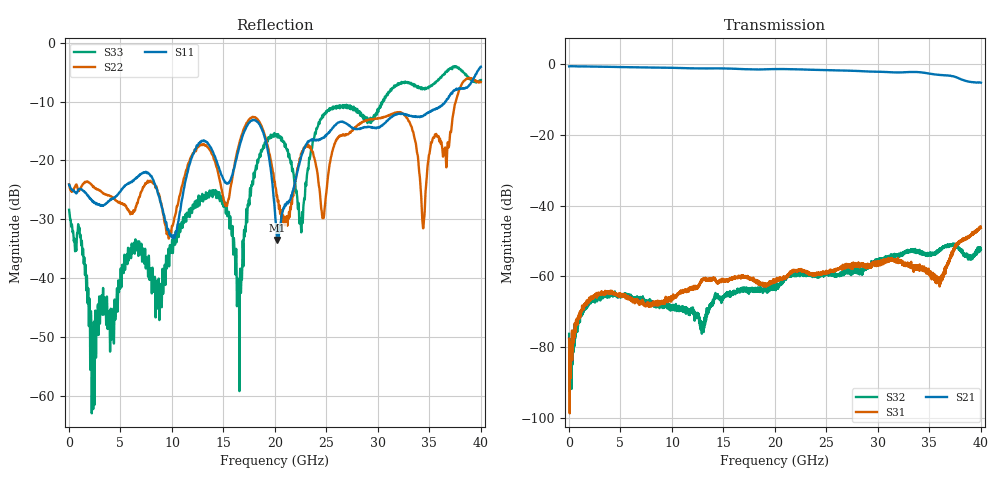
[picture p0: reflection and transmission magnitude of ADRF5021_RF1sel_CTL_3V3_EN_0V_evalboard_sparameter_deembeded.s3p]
! Device:  ADRF5021
! Description: SOI MMIC SPDT Non-Reflective Switch
! Frequency:  9 kHz -  30 GHz
! Ports:
! 	RFC	= Port 1
!	RF1	= Port 2
!	RF2	= Port 3
! Vdd:  +3.3 Volt
! Vss:  -2.5 Volt
! Control:  0/+3.3 Volt
! State:  RF1 Selected (Vctl= 3.3 V, Ven= 0 V)
! Data:	Data was collected using a calibrated network analyzer with AFR software.
!	Fixtures were calculated using AFR and fixturing was applied to collect
!	this Deembedded  S Parameter data of ADRF5021.
! Note:	Analog Devices supplies this data as a sample of measured data at the package pin
!	for this product.  Your particular data for this product may vary.
!	Data was taken at 25 degrees C.
!	Analog Devices reserves the right to change this data at anytime.
# Hz S  dB  R 50
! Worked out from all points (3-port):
!   4000 points, 10 MHz to 40 GHz, reference 50 ohm
!   strongest paths, dB at 10 MHz, 10.01 GHz, 20.01 GHz, 30.01 GHz, 40 GHz:
!     S21: -0.7, -1.1, -1.4, -2.2, -5.3
!     S31: -77.6, -66.2, -61.0, -56.4, -46.3
!     S32: -76.2, -68.1, -63.7, -55.7, -52.3
!   lowest |S11| = -33.5 dB at 20.24 GHz (marker M1), VSWR 1.04, Z = 48 + j0.696 ohm
!   |S11| at or under -10 dB: start of sweep to 36.54 GHz
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1e7  -24.09 -1.8  -0.68 -0.2  -82.91 -11.9
     -0.68 -0.1  -24.04 -2.1  -77.96 -98.2
     -77.58 63.8  -76.18 166.8  -28.37 -165.7
2.35e9  -26.90 -40.8  -0.74 -28.0  -65.82 54.0
        -0.75 -27.9  -24.50 -36.0  -66.67 35.7
        -65.82 52.2  -66.93 36.6  -62.18 -25.7
1.369e10  -17.60 -96.9  -1.26 -158.8  -60.87 81.7
          -1.26 -158.8  -18.26 -61.8  -68.81 -36.4
          -61.15 83.6  -68.45 -39.1  -25.41 -27.3
1.65e10  -17.95 -114.9  -1.41 167.7  -60.45 81.0
         -1.41 167.8  -17.35 -130.6  -63.86 -85.8
         -60.32 80.7  -64.08 -85.6  -41.36 161.6
2.001e10  -29.40 -157.0  -1.45 127.0  -61.15 70.3
          -1.45 127.1  -24.04 -105.2  -63.24 -118.8
          -60.98 68.0  -63.66 -119.9  -15.87 -29.3
2.024e10  -33.47 160.0  -1.44 124.2  -61.00 71.5
          -1.44 124.2  -26.46 -100.9  -62.76 -122.0
          -60.69 66.3  -63.34 -121.6  -16.09 -23.8
2.254e10  -19.37 -177.7  -1.54 95.0  -58.08 66.2
          -1.55 95.1  -18.84 -171.7  -59.65 -160.2
          -58.47 67.6  -59.37 -161.8  -31.75 -46.8
2.995e10  -14.39 -102.0  -2.21 1.8  -56.40 -1.8
          -2.21 1.9  -12.84 -86.6  -55.69 109.1
          -56.57 -5.2  -56.01 104.6  -11.45 -106.1
3.441e10  -12.43 -107.0  -2.46 -58.7  -57.85 5.0
          -2.46 -58.6  -31.44 8.6  -53.32 29.1
          -58.31 1.2  -53.24 29.9  -7.81 -111.1
4e10  -4.09 -123.0  -5.27 -146.9  -46.06 11.0
      -5.29 -146.8  -6.67 -37.7  -51.94 -92.1
      -46.28 11.6  -52.25 -92.0  -6.35 -147.8
